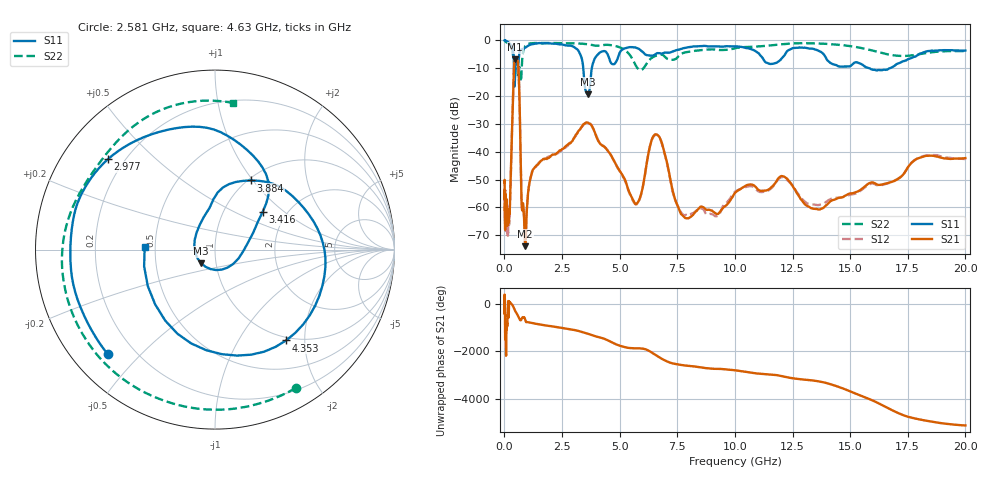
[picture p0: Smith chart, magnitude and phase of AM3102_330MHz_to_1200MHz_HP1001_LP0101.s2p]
! Date/Time: Tue, Sep 11, 2018 5:18 PM
! Network Analyzer: Agilent Technologies E8362B Rev: A.07.50.63
! Sweep from 0.010 to 20.000 GHz, 1601 Points, Sweep Type: LOG
! Power Supply: 4.949 V, 0.001 A
# Hz S DB R 50
!freq MagS11 AngS11 MagS21 AngS21 MagS12 AngS12 MagS22 AngS22
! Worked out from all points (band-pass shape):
!   1601 points, 10 MHz to 20 GHz, reference 50 ohm
!   highest |S21| = -6.84 dB at 464.5 MHz (marker M1); lowest = -73.9 dB at 907.7 MHz (marker M2)
!   |S21| within 3 dB of the highest: 415.4 MHz to 607.3 MHz (191.9 MHz wide, 37.5 % of centre)
!   lowest |S11| = -19.3 dB at 3.617 GHz (marker M3), VSWR 1.24, Z = 42.4 - j6.48 ohm
!   |S11| at or under -10 dB: 418.1 MHz to 470.3 MHz (52.25 MHz wide, 11.8 % of centre); 3.422 GHz to 3.791 GHz (369 MHz wide, 10.2 % of centre); 15.84 GHz to 16.71 GHz (873.1 MHz wide, 5.36 % of centre)
!   |S22| runs from -14.8 to -0.2 dB; largest |S21 - S12| = 0.007
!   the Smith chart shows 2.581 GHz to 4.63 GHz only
!   S11 on the Smith chart (normalised r, x): 2.581 GHz: 0.11, -0.40; 2.977 GHz: 0.14, +0.36; 3.416 GHz: 1.52, +0.72; 3.884 GHz: 1.03, +0.98; 4.353 GHz: 0.95, -1.63; 4.63 GHz: 0.44, +0.02
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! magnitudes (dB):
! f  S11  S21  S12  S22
! 10 MHz  0.0  -51.0  -56.3  -0.2
! 35.55 MHz  0.0  -61.3  -66.7  -0.3
! 48.41 MHz  0.0  -56.5  -54.5  -0.4
! 126.4 MHz  -0.4  -65.4  -65.0  -0.8
! 236.6 MHz  -1.1  -60.1  -59.5  -1.4
! 447.2 MHz  -16.3  -7.1  -7.1  -7.1
! 464.5 MHz  -11.6  -6.8  -6.9  -6.6
! 611.9 MHz  -7.7  -10.5  -10.6  -12.5
! 750.6 MHz  -3.1  -59.0  -58.7  -10.3
! 907.7 MHz  -2.6  -73.9  -70.5  -1.9
! 1.59 GHz  -1.0  -43.2  -43.2  -0.9
! 2.581 GHz  -1.6  -38.7  -38.8  -1.0
! 2.977 GHz  -2.1  -35.7  -35.5  -1.0
! 3.416 GHz  -9.4  -30.2  -30.5  -1.2
! 3.617 GHz  -19.3  -29.5  -29.3  -1.4
! 3.884 GHz  -7.2  -32.2  -32.2  -1.8
! 4.353 GHz  -3.8  -38.3  -38.3  -1.6
! 4.63 GHz  -8.1  -41.3  -41.3  -1.7
! 5.652 GHz  -2.5  -58.4  -58.6  -8.2
! 6.58 GHz  -4.8  -33.7  -33.9  -5.5
! 7.92 GHz  -2.5  -63.8  -62.7  -4.2
! 20 GHz  -3.6  -42.3  -42.6  -3.8
